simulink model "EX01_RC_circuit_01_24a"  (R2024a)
settings: Solver=ode45  StartTime=0.0  StopTime=10  RelTol=1e-3  EnableMultiTasking=on
libraries: spsSeriesRLCBranchLib x2, spsControlledVoltageSourceLib x1, spsGroundLib x1, spsMultimeterLib x1, spspowerguiLib x1

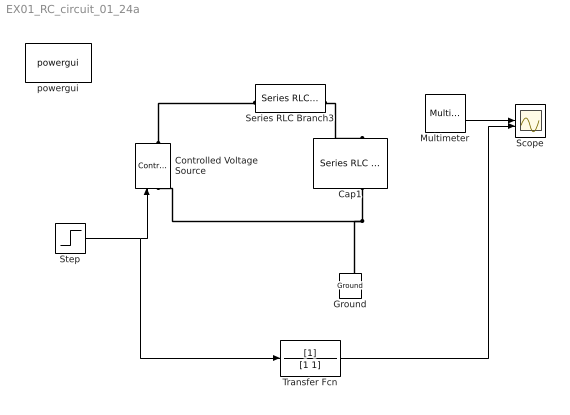
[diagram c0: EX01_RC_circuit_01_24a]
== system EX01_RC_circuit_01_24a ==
  Cap1 : spsSeriesRLCBranchLib/Series RLC Branch  LConnTagsString=__new0  RConnTagsString=__new0  BranchType=C  Resistance=10000  Inductance=1e-3  SetiL0=off  InitialCurrent=0  Capacitance=1  Setx0=off  InitialVoltage=0  Measurements=Branch voltage
  Controlled Voltage Source : spsControlledVoltageSourceLib/Controlled Voltage Source  Initialize=on  Source_Type=AC  Amplitude=0  Phase=0  Frequency=0  Measurements=Voltage
  Ground : spsGroundLib/Ground  LConnTagsString=a
  Multimeter : spsMultimeterLib/Multimeter  L=2  sel=[2 1]  yselected={}  Gain=[1 1]  OutputType=Complex  PlotAtSimulationStop=off  PhasorSimulation=off
  Scope : Scope  NumInputPorts=2
  Series RLC Branch3 : spsSeriesRLCBranchLib/Series RLC Branch  LConnTagsString=__new0  RConnTagsString=__new0  BranchType=R  Resistance=1  Inductance=1e-3  SetiL0=off  InitialCurrent=0  Capacitance=1e-6  Setx0=off  InitialVoltage=0  Measurements=None
  Step : Step  Time=0  SampleTime=0
  Transfer Fcn : TransferFcn  Denominator=[1 1]
  powergui : spspowerguiLib/powergui  Priority=1  SimulationMode=Continuous  SampleTime=50e-6  frequency=60  Iterations=50  frequencyindice=0  Pbase=100e6  ErrMax=1e-4  UnitsV=kV  UnitsW=MW  buscounter=0  FunctionMessages=off  echomessages=off  EnableUseOfTLC=off  CurrentSourceSwitches=off  DisableSnubberDevices=on  DisableRonSwitches=on  DisableVfSwitches=on  DisplayEquations=off  AutomaticDiscreteSolvers=off  SolverType=Tustin  Interpol=off  ExternalGateDelay=off  methode=off  Ts=0  x0status=blocks  SPID=on  SwTol=0  HookPort=off  NonlinearTolerance=1e-4  nMaxIteration=100  ContinueOnMaxIteration=off  RestoreLinks=warning  ResistiveCurrentMeasurement=off  Frange=[0:2:500]  Ylog=off  Xlog=on  ShowGrid=off  save=off  variable=ZData  structure=0  ZoomFFT=off  StartTime=0.0  cycles=1  DisplayStyle=1  fundamental=60  FreqAxis=off  MaxFrequency=1000  frequencyindicesteady=1  RmsSteady=1  display=off
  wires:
  Step/1 -> Controlled Voltage Source/1, Transfer Fcn/1
  Multimeter/1 -> Scope/1
  Transfer Fcn/1 -> Scope/2
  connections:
  Series RLC Branch3/RConn1 -- Cap1/LConn1
  Cap1/RConn1 -- Ground/LConn1 -- Controlled Voltage Source/LConn1
  Controlled Voltage Source/RConn1 -- Series RLC Branch3/LConn1
